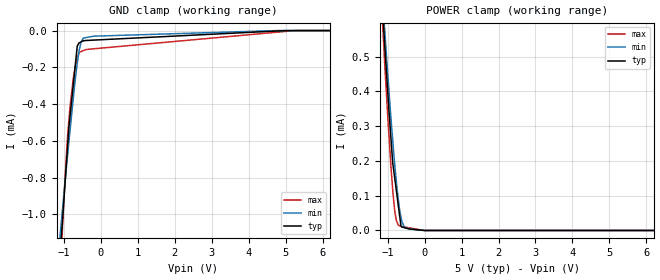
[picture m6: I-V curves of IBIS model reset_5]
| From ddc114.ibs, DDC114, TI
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|   reset_5 Model
[Model]   reset_5
Model_type   Input
Vinl = 1
Vinh = 4
|   typ   min   max
|   (nom PVT)   (fast PVT)   (slow PVT)
|C_comp from frequency sweep method (F=0.01MHz)
|Average
|C_comp   5.808e-13   4.922e-13   6.708e-13
|C_comp from LC tank measurement(L=1nH)
|Average
|Resonant Frequency(Hz)   5.879e+10   6.291e+10   4.374e+10
C_comp   7.336e-15   6.407e-15   1.325e-14
| Where nom  PVT is Nominal Process, 5V, 27C
|   Fast PVT is Strong Process,  5.25V, -40C
|   Slow PVT is Weak Process,   4.75V, 87C
[Model Spec]
|Subparameter   typ   min   max
Vinl   1.0   0.95   1.05
Vinh   4.0   3.8   4.2
[Voltage Range]   5   4.75   5.25
[Temperature Range]   27   87   -40
[Power Clamp Reference]   5   4.75   5.25
[GND Clamp Reference]   0   0   0
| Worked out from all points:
|   GND clamp passes 1 mA (typ) near -1.03 V on its own axis
|   POWER clamp passes 1 mA (typ) near -1.34 V on its own axis
[GND Clamp]
|   Voltage   I(typ)   I(min)   I(max)
-5V       -13.86mA   -10.07mA   -20.07mA
-1.088V   -1.181mA   -1.08mA    -1.282mA
-1.05V    -1.067mA   -998.1uA   -1.119mA
-897.8mV  -622.8uA   -671.4uA   -567.4uA
-865mV    -527.4uA   -606uA     -488.2uA
-834.7mV  -468uA     -545.6uA   -415uA
-745.5mV  -292.7uA   -367.3uA   -259.9uA
-640mV    -85.61uA   -179.8uA   -146.2uA
-536.7mV  -61.74uA   -63.19uA   -114.2uA
-475mV    -55.44uA   -40.68uA   -109.3uA
5.25V     0A         0A         0A
10V       0A         0A         0A
[POWER Clamp]
|   Voltage   I(typ)   I(min)   I(max)
-5V       8.363mA    7.771mA    9.163mA
-1.306V   940.2uA    948.1uA    932.4uA
-1.088V   548.1uA    588.9uA    495.6uA
-1.08V    534.6uA    576.8uA    480.2uA
-992.2mV  389.5uA    442.5uA    318.2uA
-865mV    196.5uA    262.4uA    119.3uA
-808.5mV  150.4uA    189.2uA    56.51uA
-714mV    73.15uA    91.68uA    15.68uA
-625mV    10.42uA    31.39uA    11.52uA
-536.7mV  7.781uA    7.715uA    9.897uA
-84.44fV  0A         0A         0A
10V       0A         0A         0A
